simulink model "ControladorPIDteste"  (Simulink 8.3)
settings: Solver=ode45  StartTime=0.0  StopTime=10.0  RelTol=1e-3
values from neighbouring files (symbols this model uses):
  A = 1.0    (= 1)    [ScriptDeInicializacaoPID.m]
  Kp = 3.0    (= 3)    [ScriptDeInicializacaoPID.m]    (also in sistemadecontrolePI.m = 2)
  Kw = 1.0    (= 1)    [ScriptDeInicializacaoPID.m]
  N = 100.0    (= 100)    [ScriptDeInicializacaoPID.m]
  Power = 0.0    (= 0)    [ScriptDeInicializacaoPID.m]
  T = 0.25    [ScriptDeInicializacaoPID.m]
  Td = 0.0    (= 0)    [ScriptDeInicializacaoPID.m]
  Ti = 0.2    [ScriptDeInicializacaoPID.m]    (also in sistemadecontrolePI.m = 0.1)
libraries: simulink x2

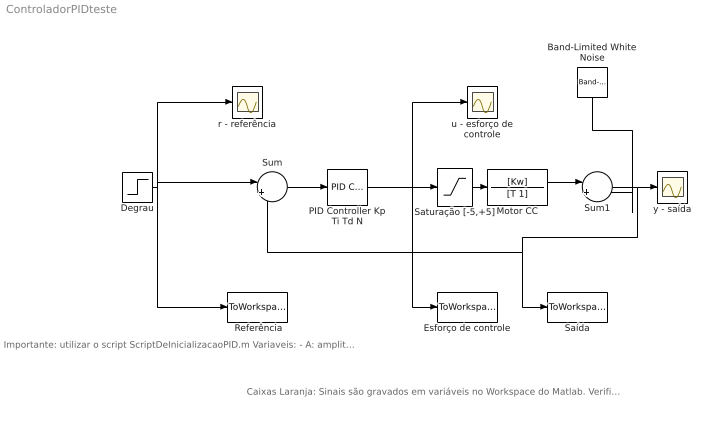
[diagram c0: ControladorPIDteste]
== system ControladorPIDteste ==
  note: Importante: utilizar o script ScriptDeInicializacaoPID.m Variaveis: - A: amplitude do degrau, - Power: potencia do sinal de ruído, Parâmetros do motor: - Kw: ganho do motor, - T: constante de tempo do motor, Parâmetros do controlador PID: - Kp: ganho proporcional, - Ti: tempo integral, - Td: tempo derivativo, - N: parâmetro do filtro de 1a. ordem
  note: Caixas Laranja: Sinais são gravados em variáveis no Workspace do Matlab. Verifique o Script PlotagraficoPID.m que plota as variáveis r,u,y
  " Referência" : ToWorkspace  VariableName=r  SampleTime=-1
  Band-Limited White Noise : simulink/Sources/Band-Limited White Noise  Cov=[Power]  Ts=0.1  seed=[23341]
  Degrau : Step  Time=0.0  After=A  SampleTime=0
  Esforço de controle : ToWorkspace  VariableName=u  SaveFormat=Structure With Time  SampleTime=-1
  Motor CC : TransferFcn  Numerator=[Kw]  Denominator=[T 1]
  PID Controller Kp Ti Td N : simulink/Continuous/PID Controller  Controller=PID  TimeDomain=Continuous-time  SampleTime=1  IntegratorMethod=Forward Euler  FilterMethod=Forward Euler  Form=Ideal  P=Kp  I=1/Ti  D=Td  N=N  InitialConditionSource=internal  InitialConditionForIntegrator=0  InitialConditionForFilter=0  ExternalReset=none  LimitOutput=off  UpperSaturationLimit=inf  LowerSaturationLimit=-inf  LinearizeAsGain=on  AntiWindupMode=none  Kb=1  TrackingMode=off  Kt=1  PParamMin=[]  PParamMax=[]  IParamMin=[]  IParamMax=[]  DParamMin=[]  DParamMax=[]  NParamMin=[]  NParamMax=[]  KbParamMin=[]  KbParamMax=[]  KtParamMin=[]  KtParamMax=[]  POutMin=[]  POutMax=[]  IOutMin=[]  IOutMax=[]  DOutMin=[]  DOutMax=[]  NOutMin=[]  NOutMax=[]  KbOutMin=[]  KbOutMax=[]  KtOutMin=[]  KtOutMax=[]  IntegratorOutMin=[]  IntegratorOutMax=[]  FilterOutMin=[]  FilterOutMax=[]  SumOutMin=[]  SumOutMax=[]  SumI1OutMin=[]  SumI1OutMax=[]  SumI2OutMin=[]  SumI2OutMax=[]  SumI3OutMin=[]  SumI3OutMax=[]  SumDOutMin=[]  SumDOutMax=[]  SaturationOutMin=[]  SaturationOutMax=[]  IntegratorContinuousStateAttributes=''  IntegratorStateMustResolveToSignalObject=off  IntegratorRTWStateStorageClass=Auto  FilterContinuousStateAttributes=''  FilterStateMustResolveToSignalObject=off  FilterRTWStateStorageClass=Auto
  Saturação [-5,+5] : Saturate  UpperLimit=5  LowerLimit=-5
  Saída : ToWorkspace  VariableName=y  SaveFormat=Structure With Time  SampleTime=-1
  Sum : Sum  Inputs=|+-
  Sum1 : Sum  Inputs=|++
  r - referência : Scope
  u - esforço de controle : Scope
  y - saída : Scope
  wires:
  Sum/1 -> PID Controller Kp Ti Td N/1
  Saturação [-5,+5]/1 -> Motor CC/1
  PID Controller Kp Ti Td N/1 -> Esforço de controle/1, u - esforço de controle/1, Saturação [-5,+5]/1
  Degrau/1 -> Sum/1, " Referência"/1, r - referência/1
  Band-Limited White Noise/1 -> Sum1/2
  Motor CC/1 -> Sum1/1
  Sum1/1 -> y - saída/1, Saída/1, Sum/2
